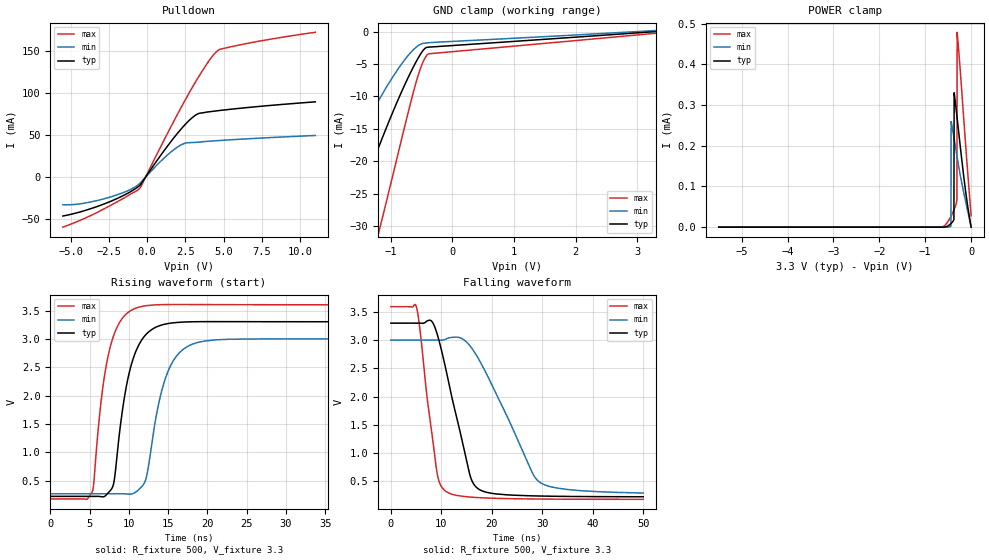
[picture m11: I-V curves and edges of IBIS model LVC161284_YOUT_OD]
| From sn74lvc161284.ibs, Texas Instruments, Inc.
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[Model]   LVC161284_YOUT_OD
Model_type  Open_drain
Enable   Active-Low
Vref =   3.3
Rref =   500
Cref =   50p
Vmeas =   1.5
| variable   typ   min   max
C_comp   3.92pF   3.60pF   4.27pF
| C_pulldown   3.37pF   3.03pF   4.14pF
| C_tri-state   3.92pF   3.60pF   4.27pF
[Temperature Range]   40   100   -40
| Ambient temperature   25   85   -40
[Voltage range]   3.3   3   3.6
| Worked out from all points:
|   slope of the pulldown table from 0 to 0.495 V, typ, clamps not added: 37.8 ohm
|   rising waveform, R_fixture 500, V_fixture 3.3: 20-80 % time 2.21ns typ, 2.5ns min, 1.98ns max; typ from 0.225 V to 3.3 V
|   falling waveform, R_fixture 500, V_fixture 3.3: 20-80 % time 4.68ns typ, 8.48ns min, 2.71ns max; typ from 3.3 V to 0.227 V
[GND Clamp]
| LVC161284_YOUT_OD
|   Voltage   I(typ)   I(min)   I(max)
-5.5V     -142.1mA   -99.43mA   -215.9mA
-2.265V   -46.37mA   -30.73mA   -74.31mA
-2.185V   -44.13mA   -29.13mA   -70.97mA
-1.685V   -30.47mA   -19.42mA   -50.47mA
-1.195V   -17.9mA    -10.67mA   -31.15mA
-1.14V    -16.57mA   -9.764mA   -29.03mA
-850mV    -9.911mA   -5.389mA   -17.74mA
-600mV    -4.914mA   -2.538mA   -8.294mA
-485mV    -3.066mA   -1.848mA   -4.955mA
-435mV    -2.546mA   -1.777mA   -3.97mA
-395mV    -2.411mA   -1.736mA   -3.499mA
3.3V      141.7pA    168.7uA    -261.4uA
[POWER Clamp]
| LVC161284_YOUT_OD
|   Voltage   I(typ)   I(min)   I(max)
-5.5V     46.85nA    131.5nA    6.203nA
-585mV    12.19nA    2.675nA    3.285uA
-440mV    8.724uA    2.432uA    26.26uA
-435mV    9.268uA    259.4uA    27.35uA
-375mV    19.07uA    220.6uA    42.01uA
-370mV    330uA      217.2uA    43.39uA
-310mV    273uA      175.6uA    67.35uA
-305mV    267.9uA    172.1uA    478.3uA
-250mV    212.1uA    135.7uA    403.5uA
-130mV    96.77uA    68.64uA    218.4uA
-70mV     47.77uA    37uA       127.7uA
-95.1fV   141.7pA    739.8pA    27.84uA
[Pulldown]
| LVC161284_YOUT_OD
|   Voltage   I(typ)   I(min)   I(max)
-5.5V     -46.7mA    -33.42mA   -59.97mA
-2.72V    -31.74mA   -25.77mA   -37.32mA
-1.275V   -19.72mA   -16.73mA   -22.76mA
-480mV    -10.32mA   -8.029mA   -13.64mA
1.565V    41.96mA    29.5mA     59.61mA
2.25V     57.29mA    38.13mA    83.15mA
2.75V     66.96mA    40.53mA    99.64mA
3.395V    75.38mA    41.18mA    119.7mA
4.12V     77.46mA    42.37mA    139.8mA
4.62V     78.59mA    43mA       150.1mA
6.93V     83.02mA    45.54mA    160mA
11V       89.16mA    49.12mA    171.9mA
[Ramp]
| LVC161284_YOUT_OD
| variable   typ   min   max
dV/dt_r   1.85/2.22E-09   1.64/2.50E-09   2.06/1.99E-09
dV/dt_f   1.88/4.77E-09   1.66/8.67E-09   2.07/2.74E-09
R_load = 500
[Rising Waveform]
| LVC161284_YOUT_OD
R_fixture =   500
C_fixture =   0
L_fixture =   0
V_fixture =   3.3
V_fixture_min = 3
V_fixture_max = 3.6
|   Time   V(typ)   V(min)   V(max)
0s        225.3mV    271.6mV    181mV
5.34ns    225.3mV    271.6mV    306.1mV
6.64ns    217.2mV    271.6mV    2.095V
7.835ns   363.7mV    271.6mV    2.959V
9.44ns    1.972V     271mV      3.406V
10.53ns   2.643V     275.1mV    3.52V
12.18ns   3.078V     537.8mV    3.584V
14.85ns   3.267V     2.38V      3.605V
17.67ns   3.3V       2.881V     3.606V
50ns      3.301V     3V         3.6V
[Falling Waveform]
| LVC161284_YOUT_OD
R_fixture =   500
C_fixture =   0
L_fixture =   0
V_fixture =   3.3
V_fixture_min = 3
V_fixture_max = 3.6
|   Time   V(typ)   V(min)   V(max)
0s        3.3V       3V         3.592V
5.065ns   3.3V       3V         3.589V
5.715ns   3.3V       3V         3.231V
7.875ns   3.349V     3V         1.521V
9.09ns    3.133V     3V         687.6mV
10.8ns    2.527V     3.013V     330.6mV
15.64ns   623.4mV    2.904V     222.6mV
17.38ns   363.4mV    2.667V     211.9mV
29.32ns   240.6mV    497.1mV    187.2mV
50ns      226.9mV    293.2mV    181.6mV
